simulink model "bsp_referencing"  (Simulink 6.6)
settings: Solver=VariableStepDiscrete  StartTime=0.0  StopTime=5.0  FixedStep=1e-2  RelTol=1e-3
model workspace: external: MAT-File (data not in the file)

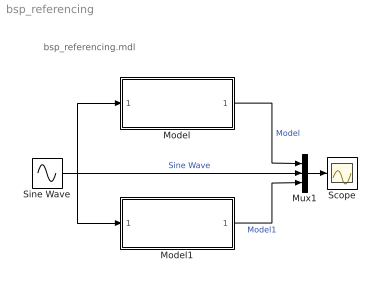
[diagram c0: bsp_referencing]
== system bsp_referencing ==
  note: bsp_referencing.mdl
  Model : ModelReference  ModelName=bsp_referencing_g  ParameterArgumentNames=gain  ParameterArgumentValues=0.1  ModelReferenceVersion=1.54  CopyOfModelName=bsp_referencing_g
  Model1 : ModelReference  ModelName=bsp_referencing_g  ParameterArgumentNames=gain  ParameterArgumentValues=0.5  ModelReferenceVersion=1.54  CopyOfModelName=bsp_referencing_g
  Mux1 : Mux  Inputs=3
  Scope : Scope
  Sine Wave : Sin  Frequency=sqrt(10)  SampleTime=0
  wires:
  Model/1 -> Mux1/1  "Model"
  Sine Wave/1 -> Model/1, Model1/1, Mux1/2  "Sine Wave"
  Mux1/1 -> Scope/1
  Model1/1 -> Mux1/3  "Model1"
